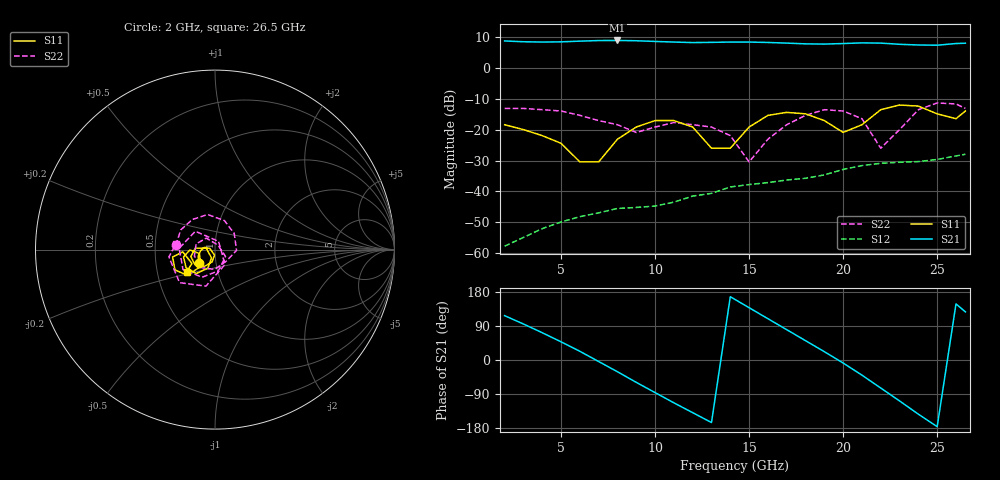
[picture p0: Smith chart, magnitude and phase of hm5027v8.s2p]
! HMMC-5027
! S-PARAMETERS at Vdd=8V; Idd=250mA.  LAST UPDATED 02-07-97
# GHZ  S  MA  R  50
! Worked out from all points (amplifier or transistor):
!   26 points, 2 GHz to 26.5 GHz, reference 50 ohm
!   highest |S21| = 8.8 dB at 8 GHz (marker M1)
!   |S21| within 3 dB of that: start of sweep to end of sweep
!   unconditionally stable (mu >= 1): start of sweep to end of sweep
!   at 6 GHz: K = 46.08, MAG = 8.8 dB, |S12| = -48.2 dB
!   at 15 GHz: K = 14.67, MAG = 8.4 dB, |S12| = -37.8 dB
!   at 26.5 GHz: K = 4.59, MAG = 8.4 dB, |S12| = -28.0 dB
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2  0.12 -140.0  2.72 117.0  0.0013 -165.0  0.22 174.0
4  0.08 -176.0  2.61 72.0  0.0025 154.0  0.21 127.0
6  0.03 167.0  2.7 23.0  0.0039 91.0  0.17 72.0
7  0.03 -95.0  2.76 -4.0  0.0045 75.0  0.14 40.0
8  0.07 -103.0  2.77 -31.0  0.0053 21.0  0.12 -2.0
9  0.11 -122.0  2.74 -59.0  0.0055 10.0  0.09 -47.0
10  0.14 -143.0  2.67 -86.0  0.0058 -16.0  0.11 -91.0
11  0.14 -164.0  2.61 -113.0  0.0067 -33.0  0.13 -130.0
13  0.05 170.0  2.58 -165.0  0.0093 -76.0  0.11 163.0
14  0.05 -113.0  2.61 167.0  0.0118 -96.0  0.08 127.0
15  0.11 -111.0  2.61 138.0  0.0129 -125.0  0.03 57.0
16  0.17 -128.0  2.57 109.0  0.0139 -149.0  0.07 -33.0
17  0.19 -148.0  2.51 80.0  0.0153 -175.0  0.12 -81.0
19  0.14 -179.0  2.42 22.0  0.0185 142.0  0.21 -148.0
20  0.09 -166.0  2.47 -8.0  0.0227 113.0  0.2 178.0
21  0.12 -130.0  2.53 -40.0  0.0262 81.0  0.15 137.0
22  0.21 -137.0  2.51 -74.0  0.0285 43.0  0.05 67.0
23  0.25 -153.0  2.4 -108.0  0.0296 13.0  0.1 -56.0
24  0.24 -170.0  2.34 -143.0  0.0304 -16.0  0.21 -104.0
25  0.18 -176.0  2.32 -176.0  0.0329 -45.0  0.27 -137.0
26  0.15 -149.0  2.47 148.0  0.0375 -78.0  0.26 -171.0
26.5  0.2 -142.0  2.5 127.0  0.0399 -99.0  0.22 172.0
